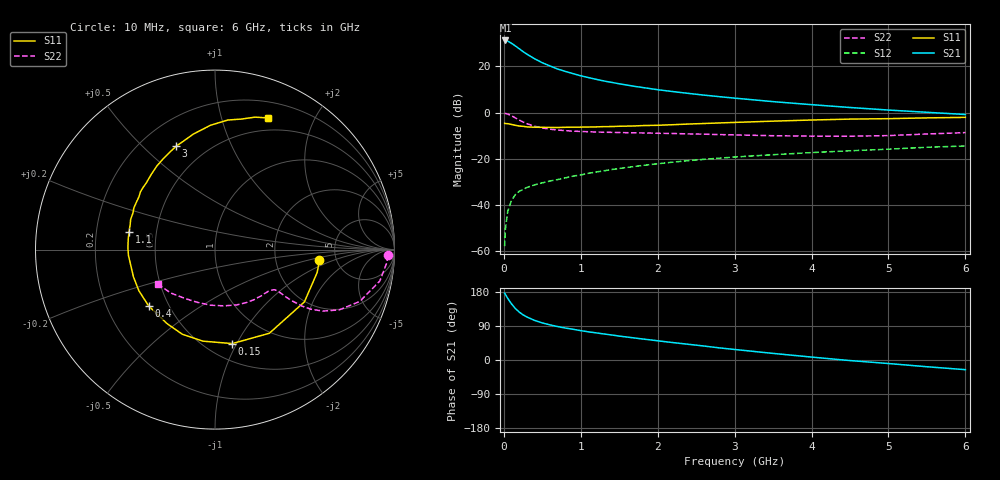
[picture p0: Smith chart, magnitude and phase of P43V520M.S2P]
! SIEMENS Small Signal Semiconductors
! BFP182
! Si NPN RF Bipolar Junction Transistor in SOT143
! VCE = 3.5 V  IC = 20 mA
! Common Emitter S-Parameters:  March  1996
# GHz  S  MA  R  50
!  f  S11  S21  S12  S22
! GHz  MAG  ANG  MAG  ANG  MAG  ANG  MAG  ANG
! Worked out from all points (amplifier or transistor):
!   36 points, 10 MHz to 6 GHz, reference 50 ohm
!   highest |S21| = 31.2 dB at 20 MHz (marker M1)
!   |S21| within 3 dB of that: start of sweep to 175.8 MHz
!   unconditionally stable (mu >= 1): 768.4 MHz to 5.343 GHz
!   at 250 MHz: K = 0.50, MSG = 29.8 dB, |S12| = -33.2 dB
!   at 1.4 GHz: K = 1.16, MAG = 16.4 dB, |S12| = -24.6 dB
!   at 6 GHz: K = 0.93, MSG = 6.8 dB, |S12| = -14.4 dB
!   S11 on the Smith chart (normalised r, x): 10 MHz: 3.69, -0.66; 150 MHz: 0.66, -0.96; 400 MHz: 0.39, -0.32; 1.1 GHz: 0.35, +0.09; 3 GHz: 0.34, +0.64; 6 GHz: 0.36, +1.42
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0.01  0.5849 -5.8  36.25 176.3  0.0013 80.3  0.9631 -1.9
0.02  0.5834 -12.6  36.35 173.3  0.003 85.9  0.9609 -4.2
0.05  0.5771 -30.3  35.23 162.8  0.0073 82.6  0.9348 -10.8
0.1  0.5558 -57.0  31.51 148.0  0.0127 67.0  0.8567 -19.7
0.15  0.5324 -79.6  27.67 135.8  0.017 60.4  0.7691 -25.9
0.2  0.5145 -97.5  24.04 126.5  0.02 56.3  0.6913 -29.7
0.25  0.5056 -111.1  20.85 119.1  0.0218 53.4  0.6281 -31.9
0.3  0.4915 -122.8  18.36 113.5  0.0242 51.9  0.5776 -33.0
0.4  0.4848 -139.8  14.62 104.4  0.0275 50.6  0.5088 -33.7
0.5  0.4822 -151.6  11.98 97.9  0.0304 49.7  0.4666 -33.7
0.6  0.4792 -161.6  10.21 92.7  0.0333 50.7  0.4395 -33.5
0.7  0.4773 -169.5  8.771 88.2  0.0358 52.2  0.4215 -33.5
0.9  0.4855 178.9  6.975 81.0  0.0425 52.9  0.3985 -34.1
1.1  0.4892 168.4  5.731 74.3  0.0489 53.7  0.3867 -35.8
1.5  0.5081 152.9  4.206 63.1  0.0621 53.4  0.3723 -40.2
1.8  0.5253 142.3  3.503 55.5  0.0721 52.1  0.3649 -44.7
2.2  0.549 130.3  2.85 45.9  0.0852 49.6  0.3544 -51.7
3  0.6151 110.6  2.06 27.8  0.1099 42.9  0.3309 -68.6
3.5  0.6553 100.5  1.73 17.4  0.1234 38.5  0.3173 -81.0
4.5  0.7253 84.4  1.292 -1.5  0.15 30.0  0.3099 -108.5
5.5  0.7708 73.2  1.018 -17.8  0.1786 21.9  0.3458 -135.8
6  0.7908 68.1  0.912 -25.5  0.1903 16.9  0.3706 -148.4
